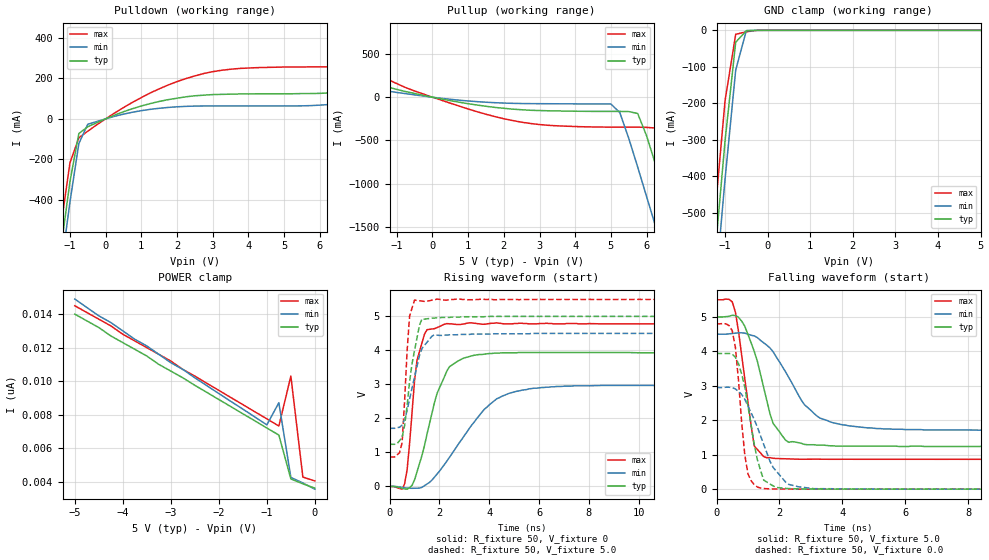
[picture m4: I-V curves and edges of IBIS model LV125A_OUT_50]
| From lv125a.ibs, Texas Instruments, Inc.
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|   Model LV125A_OUT_50
[Model]   LV125A_OUT_50
Model_type  3-state
Polarity   Non-Inverting
Enable   Active-Low
Vmeas = 2.5v
Cref = 15pf
| variable   typ   min   max
C_comp   6.5pf   4.87pf   8.13pf
[Temperature Range]   25   85   -40
[Voltage Range]   5.0   4.5   5.5
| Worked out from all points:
|   slope of the pulldown table from 0 to 0.75 V, typ, clamps not added: 14.9 ohm
|   slope of the pullup table from 0 to 0.75 V, typ, clamps not added: 13 ohm
|   GND clamp passes 1 mA (typ) near -0.46 V on its own axis
|   rising waveform, R_fixture 50, V_fixture 0: 20-80 % time 905ps typ, 1.82ns min, 381ps max; typ from 0 V to 3.93 V
|   falling waveform, R_fixture 50, V_fixture 5.0: 20-80 % time 670ps typ, 1.19ns min, 409ps max; typ from 5 V to 1.24 V
|   rising waveform, R_fixture 50, V_fixture 5.0: 20-80 % time 430ps typ, 530ps min, 217ps max; typ from 1.24 V to 5 V
|   falling waveform, R_fixture 50, V_fixture 0.0: 20-80 % time 472ps typ, 813ps min, 277ps max; typ from 3.94 V to 0 V
[Pulldown]
|   Voltage   I(typ)   I(min)   I(max)
-5V       -5.91A     -6A        -5.81A
-1.25V    -637mA     -741mA     -528mA
-1V       -311mA     -412mA     -218mA
-750mV    -72.6mA    -122mA     -93.4mA
-500mV    -38.8mA    -26.5mA    -60.9mA
250mV     18.5mA     12.6mA     28.5mA
1.5V      85.9mA     52.2mA     148mA
2.75V     117mA      63.7mA     224mA
3.75V     123mA      63.9mA     249mA
7V        144mA      83.2mA     274mA
8V        176mA      104mA      321mA
10V       253mA      153mA      454mA
[Pullup]
|   Voltage   I(typ)   I(min)   I(max)
-5V       431mA      240mA      803mA
-3.5V     340mA      193mA      622mA
1.5V      -105mA     -57.9mA    -197mA
3V        -154mA     -74.8mA    -316mA
5V        -164mA     -78.3mA    -346mA
5.25V     -164mA     -179mA     -346mA
5.75V     -188mA     -807mA     -346mA
6.25V     -776mA     -1.49A     -356mA
6.5V      -1.12A     -1.84A     -498mA
6.75V     -1.46A     -2.19A     -820mA
7.25V     -2.16A     -2.89A     -1.51A
10V       -6.05A     -6.78A     -5.4A
[GND Clamp]
|   Voltage   I(typ)   I(min)   I(max)
-5V       -5.91A     -6A        -5.81A
-1.5V     -974mA     -1.08A     -863mA
-1.25V    -633mA     -739mA     -520mA
-1V       -303mA     -408mA     -193mA
-750mV    -32.5mA    -109mA     -10.9mA
-500mV    -1.18mA    -669uA     -3.99mA
-250mV    -36.9nA    -297nA     -155uA
5V        3.61nA     4.25nA     3.57nA
[POWER Clamp]
|   Voltage   I(typ)   I(min)   I(max)
-5V       14nA       14.9nA     14.5nA
-4.5V     13.2nA     13.9nA     13.7nA
-4.25V    12.7nA     13.5nA     13.3nA
-4V       12.3nA     13nA       12.8nA
-3.5V     11.5nA     12.1nA     12nA
-3V       10.6nA     11.1nA     11.2nA
-2.75V    10.2nA     10.7nA     10.7nA
-1V       7.2nA      7.39nA     7.75nA
-750mV    6.78nA     8.71nA     7.32nA
-500mV    4.16nA     4.25nA     10.3nA
-250mV    3.87nA     3.92nA     4.27nA
0V        3.61nA     3.55nA     4.04nA
[Ramp]
| variable   typ   min   max
dV/dt_r   2.36E+00/8.43E-10   1.79E+00/1.80E-09   2.87E+00/3.70E-10
dV/dt_f   2.29E+00/6.65E-10   1.70E+00/1.16E-09   2.52E+00/4.24E-10
R_load = 50
[Rising Waveform]
R_fixture = 50
V_fixture = 0
|   Time   V(typ)   V(min)   V(max)
0s        0V         0V         0V
600ps     -73.6mV    -40mV      76.8mV
700ps     -78.6mV    -47.3mV    490mV
1.1ns     436mV      -49.6mV    3.72V
1.4ns     1.21V      25.2mV     4.48V
1.9ns     2.73V      363mV      4.67V
2.3ns     3.4V       749mV      4.79V
4ns       3.91V      2.4V       4.79V
5.8ns     3.94V      2.89V      4.78V
25ns      3.93V      2.97V      4.78V
[Falling Waveform]
R_fixture = 50
V_fixture = 5.0
V_fixture_min = 4.5
V_fixture_max = 5.5
|   Time   V(typ)   V(min)   V(max)
0s        5V         4.5V       5.5V
500ps     5.05V      4.52V      5.44V
700ps     4.99V      4.54V      4.58V
1.2ns     4V         4.45V      1.25V
1.6ns     2.57V      4.18V      913mV
1.8ns     1.91V      3.99V      897mV
2.3ns     1.36V      3.24V      879mV
3.2ns     1.28V      2.12V      871mV
4.2ns     1.25V      1.84V      869mV
25ns      1.24V      1.71V      866mV
[Rising Waveform]
R_fixture = 50
V_fixture = 5.0
V_fixture_min = 4.5
V_fixture_max = 5.5
|   Time   V(typ)   V(min)   V(max)
0s        1.24V      1.71V      866mV
400ps     1.35V      1.74V      995mV
500ps     1.44V      1.81V      1.29V
700ps     2.37V      2.23V      3.98V
800ps     3.08V      2.57V      5.01V
1ns       4V         3.22V      5.48V
1.2ns     4.75V      3.86V      5.46V
1.3ns     4.93V      4.06V      5.45V
1.8ns     4.95V      4.46V      5.49V
25ns      5V         4.5V       5.5V
[Falling Waveform]
R_fixture = 50
V_fixture = 0.0
|   Time   V(typ)   V(min)   V(max)
0s        3.94V      2.95V      4.8V
500ps     3.92V      2.95V      4.6V
600ps     3.83V      2.91V      4.12V
900ps     2.96V      2.61V      994mV
1ns       2.41V      2.41V      444mV
1.4ns     547mV      1.55V      34.3mV
1.8ns     95.8mV     632mV      6.22mV
2.2ns     23.5mV     202mV      4.08mV
3.1ns     5.33mV     14.2mV     2.29mV
25ns      54.8uV     59.2uV     50.7uV
